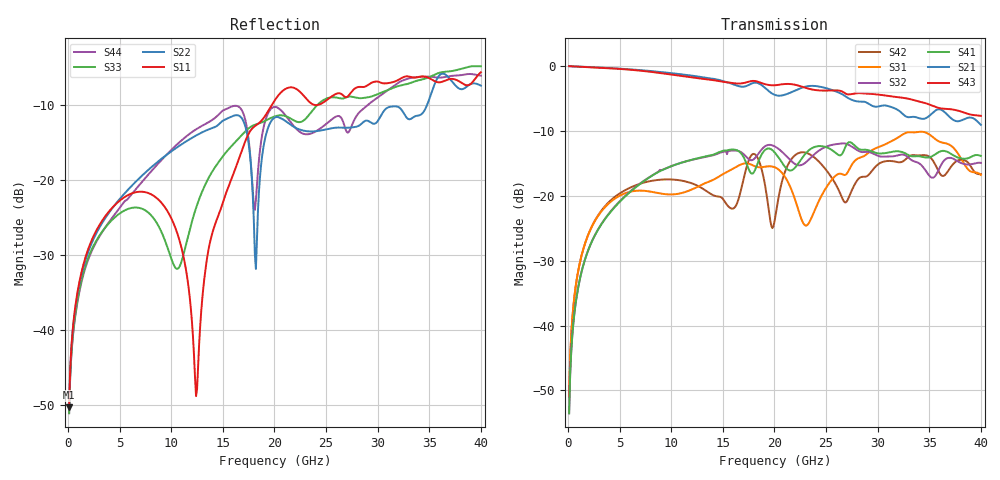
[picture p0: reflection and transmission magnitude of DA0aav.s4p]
! ADC12DJ2700AAV, ADC12DJ3200AAV, ADC08DJ3200AAV
! 144 pin AAV package
! Texas Instruments 4/21/2021
! Single-ended  S-parameters
! PORT#  PORT_NAME  NET_NAME
! PORT1:  DAxN.DIEBUMP DAxN
! PORT2:  DAxN.BGA  DAxN
! PORT3:  DAxP.DIEBUMP DAxP
! PORT4:  DAxP.BGA  DAxP
! Touchstone Ver. 1.0
! Number of ports is 4
# Hz	S	MA	R	50.000000
! SCATTERING PARAMETERS  :
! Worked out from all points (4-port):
!   400 points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, 100 MHz to 40 GHz, reference 50 ohm
!   strongest paths, dB at 100 MHz, 10.1 GHz, 20.1 GHz, 30.1 GHz, 40 GHz:
!     S43: 0.0, -1.3, -3.0, -4.4, -7.7
!     S21: 0.0, -1.1, -4.5, -6.2, -9.1
!     S41: -53.5, -15.4, -13.5, -13.5, -13.9
!     S32: -53.5, -15.4, -12.5, -13.9, -14.9
!     S31: -51.0, -19.8, -15.7, -12.5, -16.8
!     S42: -51.0, -17.5, -23.0, -15.1, -16.6
!   lowest |S11| = -50.2 dB at 100 MHz (marker M1), VSWR 1.01, Z = 50.2 + j0.261 ohm
!   |S11| at or under -10 dB: start of sweep to 19.74 GHz; 23.99861 GHz to 24.02386 GHz (25.26 MHz wide, 0.105 % of centre)
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1e8  0.003079 57.5  0.9981 -1.4  0.002828 85.3  0.002107 -95.1
     0.9981 -1.4  0.003062 57.5  0.002107 -95.1  0.002827 86.0
     0.002828 85.3  0.002107 -95.1  0.002818 55.9  0.9982 -1.3
     0.002107 -95.1  0.002827 86.0  0.9982 -1.3  0.002804 55.8
2.1e9  0.03703 41.2  0.9822 -27.0  0.05339 49.9  0.04076 -124.7
       0.9822 -27.0  0.03542 52.2  0.04086 -124.1  0.05363 65.8
       0.05339 49.9  0.04086 -124.1  0.03228 37.0  0.9807 -26.3
       0.04076 -124.7  0.05363 65.8  0.9807 -26.3  0.03145 45.3
8.9e9  0.07257 -80.7  0.9012 -111.8  0.1044 -102.3  0.1547 137.2
       0.9012 -111.8  0.1362 -15.7  0.1585 138.4  0.133 8.9
       0.1044 -102.3  0.1585 138.4  0.0475 -107.6  0.8842 -108.3
       0.1547 137.2  0.133 8.9  0.8842 -108.3  0.1328 -22.0
1.24e10  0.00365 147.3  0.8349 -154.8  0.1157 152.2  0.1934 84.3
         0.8349 -154.8  0.1983 -55.1  0.1925 86.3  0.1211 -22.3
         0.1157 152.2  0.1925 86.3  0.06529 57.4  0.8088 -148.0
         0.1934 84.3  0.1211 -22.3  0.8088 -148.0  0.218 -64.5
1.82e10  0.2317 -28.2  0.745 138.2  0.1677 27.6  0.164 12.1
         0.745 138.2  0.02564 27.7  0.1991 10.8  0.2056 37.4
         0.1677 27.6  0.1991 10.8  0.2351 -46.8  0.7646 148.8
         0.164 12.1  0.2056 37.4  0.7646 148.8  0.07378 -127.2
2.05e10  0.376 -62.8  0.5908 114.9  0.157 -28.1  0.1922 -36.6
         0.5908 114.9  0.2604 -162.3  0.2267 -34.6  0.1072 133.6
         0.157 -28.1  0.2267 -34.6  0.2706 -76.0  0.7199 124.5
         0.1922 -36.6  0.1072 133.6  0.7199 124.5  0.2972 165.3
4e10  0.5231 33.2  0.3526 -112.5  0.1449 -12.9  0.2028 67.4
      0.3526 -112.5  0.4263 -84.8  0.1795 75.9  0.1471 2.4
      0.1449 -12.9  0.1795 75.9  0.5735 65.0  0.4134 -100.1
      0.2028 67.4  0.1471 2.4  0.4134 -100.1  0.4964 -99.2
